VAR_GLOBAL CONSTANT
	
    // signals
	cOversamples 		: UDINT 	:= 10;				// number of oversamples for vibration signal
	cSampleRateVib 		: UDINT 	:= 10000;           // sample rate of vibration signal (10 samples every 1 ms)
	cSampleRatePos 		: UDINT 	:= 1000;            // sample rate of position signal  (1 sample every 1 ms) 
	cBufferLengthVib	: UDINT		:= 1000;			// buffer size of vibration signal (cWindowLength/2)
	cBufferLengthPos	: UDINT		:= 100;				// buffer size of position signal (cBufferLengthVib/cOversamples)
	
	// power spectrum settings
	cWindowLength		: UDINT		:= 2000;			// windowlength for fft calculation
	cFFTLength			: UDINT		:= 2048;			// length of FFT for mag. spectrum (order of 2 and larger than cWindowLength)
	cFFTResult 			: UDINT 	:= 1025;			// result of power spectrum (cFFTLength/2+1)
		
	// additional characteristics of rotating device
	cShaftPerimeter 	: LREAL 	:= 2 * pi * 15;		// r = 15mm
	cMinRPM 			: UDINT 	:= 400;             // definition of a minimum rotation speed  
	cMaxRPM 			: UDINT 	:= 2300;            // definition of a maximum rotation speed -> only in this segment we will calculate the order spectrum
END_VAR
